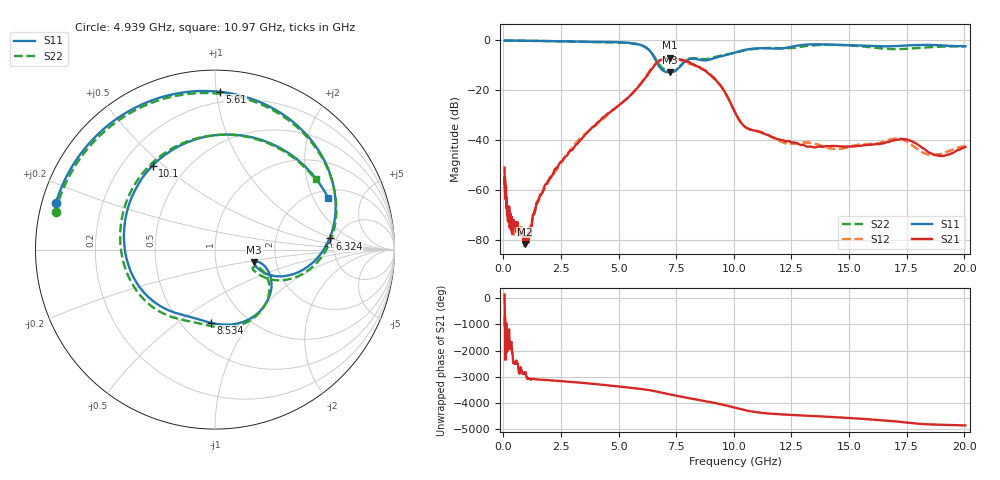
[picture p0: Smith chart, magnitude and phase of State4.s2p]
# Hz S DB R 50
!freq MagS11 AngS11 MagS21 AngS21 MagS12 AngS12 MagS22 AngS22
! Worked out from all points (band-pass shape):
!   1601 points, 50 MHz to 20.05 GHz, reference 50 ohm
!   highest |S21| = -6.95 dB at 7.237 GHz (marker M1); lowest = -81.8 dB at 922 MHz (marker M2)
!   |S21| within 3 dB of the highest: 6.561 GHz to 8.321 GHz (1.759 GHz wide, 23.6 % of centre)
!   lowest |S11| = -12.8 dB at 7.237 GHz (marker M3), VSWR 1.60, Z = 77 - j11.2 ohm
!   |S11| at or under -10 dB: 6.732 GHz to 7.707 GHz (974.7 MHz wide, 13.5 % of centre)
!   |S22| runs from -12.6 to 0.0 dB; largest |S21 - S12| = 0.027
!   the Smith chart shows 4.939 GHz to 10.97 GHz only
!   S11 on the Smith chart (normalised r, x): 4.939 GHz: 0.04, +0.14; 5.61 GHz: 0.13, +1.02; 6.324 GHz: 4.37, +0.93; 8.534 GHz: 0.69, -0.67; 10.1 GHz: 0.32, +0.46; 10.97 GHz: 2.39, +2.64
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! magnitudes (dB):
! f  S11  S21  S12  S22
! 50 MHz  0.0  -51.1  -57.7  0.0
! 108.6 MHz  0.0  -59.7  -62.3  0.0
! 135.9 MHz  0.0  -66.0  -65.3  0.0
! 218.8 MHz  0.0  -72.4  -73.4  0.0
! 250.4 MHz  0.0  -67.1  -71.0  0.0
! 274.9 MHz  0.0  -74.8  -71.6  0.0
! 308.8 MHz  0.0  -70.5  -72.9  0.0
! 369.6 MHz  0.0  -76.2  -73.9  0.0
! 608.4 MHz  -0.1  -73.6  -75.2  -0.1
! 922 MHz  -0.1  -81.8  -82.2  -0.1
! 1.005 GHz  -0.1  -79.3  -81.9  -0.1
! 2.722 GHz  -0.3  -46.5  -46.3  -0.4
! 4.939 GHz  -0.7  -26.5  -26.5  -0.8
! 5.61 GHz  -1.1  -21.1  -21.2  -1.2
! 6.324 GHz  -3.9  -12.9  -12.5  -3.9
! 7.237 GHz  -12.8  -7.0  -7.1  -12.6
! 7.402 GHz  -12.5  -7.0  -7.2  -12.4
! 8.534 GHz  -7.8  -10.9  -10.9  -7.4
! 10.1 GHz  -4.7  -29.8  -29.9  -4.7
! 10.97 GHz  -3.2  -36.4  -36.2  -3.3
! 14.37 GHz  -1.7  -42.4  -43.7  -1.8
! 20.05 GHz  -2.3  -42.8  -42.4  -2.3
